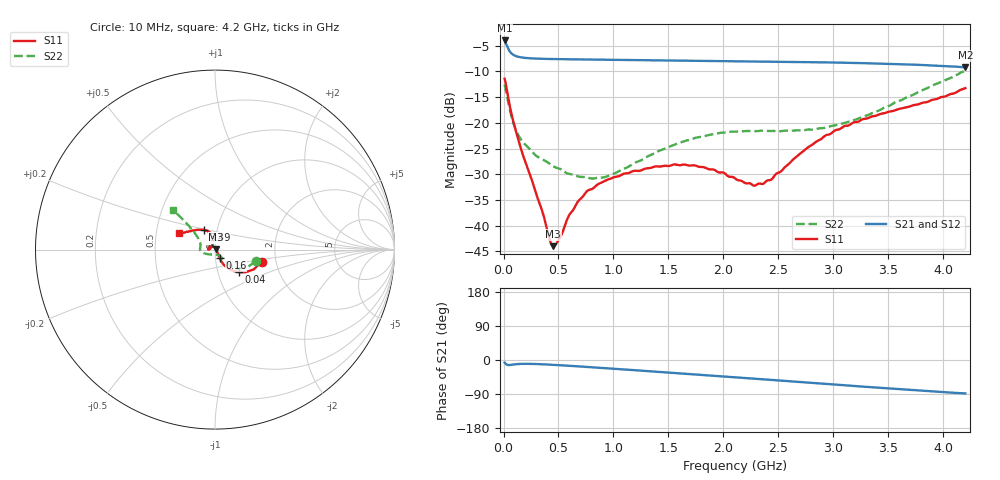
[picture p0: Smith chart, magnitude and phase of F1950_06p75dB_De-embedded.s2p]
! Integrated Device Technology
! Corporate Headquarters
! 6024 Silver Creek Valley Road
! San Jose, CA 95138  USA
! Phone:  1-408-284-8200
! Toll Free:  1-800-223-1366
! Webpage:  http://www.idt.com/
! Timing and RF Division
! 515 Groton Road, Suite 102
! Westford, MA 01886-6024
! Device:  F1950
! Description: 7-bit 0.25 dB Digital Step Attenuator
! Frequency:  150.0 -  4000.00 MHz
! Package:  4x4 mm Thin QFN Plastic Package: 24 pin
! Ports:  2 RF, 12 DC
!  Pin  1  = D0
!  Pin  2  = VDD
!  Pin  3  = Vmode
!  Pin  4  = GND
!  Pin  5  = RF1  =  Port 1
!  Pin  6  = GND
!  Pin  7  = GND
!  Pin  8  = GND
!  Pin  9  = GND
!  Pin 10  = GND
!  Pin 11  = GND
!  Pin 12  = GND
!  Pin 13  = GND
!  Pin 14  = RF2  =  Port 2
!  Pin 15  = GND
!  Pin 16  = LE
!  Pin 17  = CLK
!  Pin 18  = DATE
!  Pin 19  = D6
!  Pin 20  = D5
!  Pin 21  = D4
!  Pin 22  = D3
!  Pin 23  = D2
!  Pin 24  = D1
! State:  27
! Atten State:  6.75 dB
! Voltage:  +5.00 Volts
! Current:  Not Measured mA
! Data:  The device was measured on a the F195X evaluation board which has
!  individual transmission lines to the RF pins.  Data was collected
!  using a calibrated network analyzer.  The evaluation board was
!  de-embedded using a TRL calibration technique.
!  The reference plane is the edge of the package pin.
! Misc:  Board 2019
!  Action Tracker AT0250
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# GHz S dB R 50
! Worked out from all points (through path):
!   420 points, 10 MHz to 4.2 GHz, reference 50 ohm
!   highest |S21| = -3.96 dB at 10 MHz (marker M1); lowest = -9.2 dB at 4.2 GHz (marker M2)
!   group delay of S21, straight-line fit = 55.8 ps
!   lowest |S11| = -44.0 dB at 450 MHz (marker M3), VSWR 1.01, Z = 50.6 + j0.231 ohm
!   |S11| at or under -10 dB: start of sweep to end of sweep
!   |S22| runs from -30.8 to -9.8 dB; largest |S21 - S12| = 0.00054
!   S11 on the Smith chart (normalised r, x): 10 MHz: 1.68, -0.24; 40 MHz: 1.26, -0.33; 160 MHz: 1.05, -0.10; 3.49 GHz: 0.86, +0.19; 4.2 GHz: 0.66, +0.13
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0.01  -11.42 -14.6  -3.96 -6.7  -3.96 -6.7  -12.55 -16.1
0.04  -14.72 -43.2  -5.48 -13.2  -5.48 -13.2  -15.67 -39.5
0.1  -20.61 -60.3  -6.89 -11.6  -6.89 -11.6  -20.71 -48.0
0.16  -25.13 -61.0  -7.25 -10.3  -7.25 -10.3  -23.26 -50.0
0.35  -37.03 -36.7  -7.53 -11.2  -7.53 -11.2  -27.03 -54.4
0.42  -42.70 -5.3  -7.57 -12.2  -7.56 -12.2  -27.93 -55.7
0.45  -43.97 21.2  -7.58 -12.7  -7.58 -12.7  -28.39 -57.8
0.5  -42.81 64.7  -7.60 -13.5  -7.59 -13.5  -28.84 -61.5
0.59  -38.23 98.8  -7.62 -15.1  -7.62 -15.1  -29.88 -67.8
0.71  -34.59 116.3  -7.65 -17.4  -7.65 -17.4  -30.52 -80.0
0.77  -33.11 121.2  -7.67 -18.5  -7.67 -18.5  -30.67 -86.6
0.93  -31.17 134.5  -7.71 -21.7  -7.71 -21.7  -30.50 -108.3
1.41  -28.49 166.3  -7.82 -31.3  -7.82 -31.3  -25.48 -152.9
1.74  -28.27 179.3  -7.89 -38.1  -7.89 -38.1  -22.94 -166.8
2.11  -30.87 172.3  -7.99 -45.8  -7.98 -45.9  -21.69 -177.9
2.28  -32.22 148.9  -8.03 -49.3  -8.03 -49.4  -21.60 177.6
2.36  -31.84 135.8  -8.05 -51.0  -8.05 -51.0  -21.51 175.4
2.81  -24.20 99.9  -8.19 -60.5  -8.18 -60.5  -21.32 159.8
3.1  -20.60 105.2  -8.30 -66.7  -8.29 -66.7  -20.02 150.7
3.49  -17.91 120.0  -8.50 -74.9  -8.50 -74.9  -16.80 141.2
3.51  -17.79 121.2  -8.51 -75.3  -8.51 -75.3  -16.65 140.7
4.2  -13.23 155.5  -9.19 -88.2  -9.19 -88.3  -9.83 136.5
